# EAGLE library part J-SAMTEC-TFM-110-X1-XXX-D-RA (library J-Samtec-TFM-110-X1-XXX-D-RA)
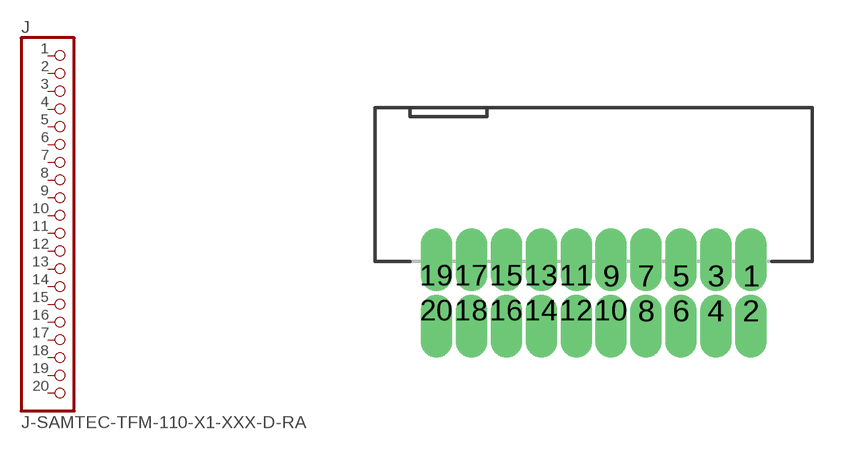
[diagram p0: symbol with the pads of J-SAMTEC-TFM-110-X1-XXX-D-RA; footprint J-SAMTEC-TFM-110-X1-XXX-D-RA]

Designator prefix J

## J-SAMTEC-TFM-110-X1-XXX-D-RA  [J-SAMTEC-TFM-110-X1-XXX-D-RA]
1  1  pas
2  2  pas
3  3  pas
4  4  pas
5  5  pas
6  6  pas
7  7  pas
8  8  pas
9  9  pas
10  10  pas
11  11  pas
12  12  pas
13  13  pas
14  14  pas
15  15  pas
16  16  pas
17  17  pas
18  18  pas
19  19  pas
20  20  pas

## Footprint J-SAMTEC-TFM-110-X1-XXX-D-RA (pad centres in mm)
drill 0.635 pad 0.965 offset: 1 5.715,0.635; 2 5.715,-0.635; 3 4.445,0.635; 4 4.445,-0.635; 5 3.175,0.635; 6 3.175,-0.635; 7 1.905,0.635; 8 1.905,-0.635; 9 0.635,0.635; 10 0.635,-0.635; 11 -0.635,0.635; 12 -0.635,-0.635; 13 -1.905,0.635; 14 -1.905,-0.635; 15 -3.175,0.635; 16 -3.175,-0.635; 17 -4.445,0.635; 18 -4.445,-0.635; 19 -5.715,0.635; 20 -5.715,-0.635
